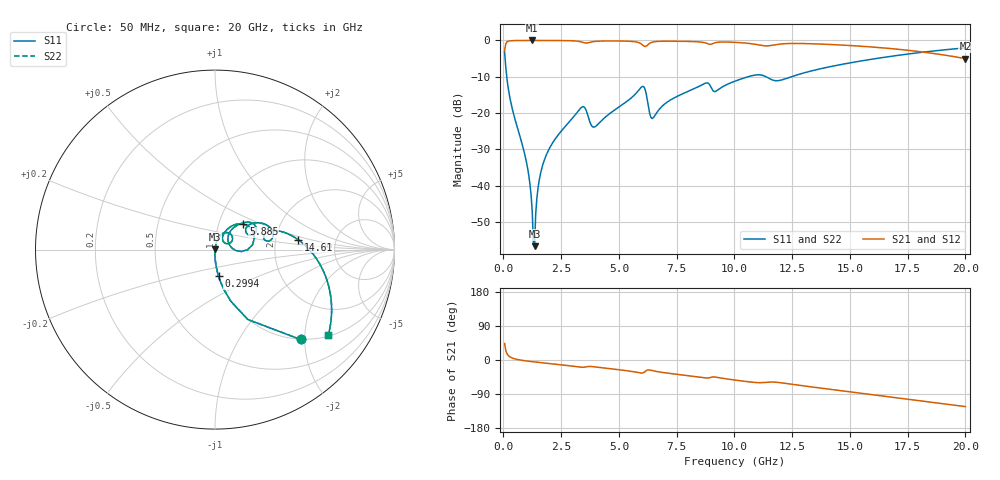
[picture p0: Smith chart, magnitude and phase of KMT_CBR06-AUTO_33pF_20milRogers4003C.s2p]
! Data measured by Modelithics Inc. support@modelithics.com 813-866-6335
! KEMET CBR06-AUTO 33pF, Pad Width= 0.851mm, Pad Length= 0.64mm, Pad Gap= 0.62mm, 20mil Rogers 4003C substrate Data, January 2022
# hz S ma R 50
! 2 Port Network Data from SP1.SP block
! freq  magS11  angS11  magS21  angS21  magS12  angS12  magS22  angS22
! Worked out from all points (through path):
!   401 points, 50 MHz to 20 GHz, reference 50 ohm
!   highest |S21| = -0.01 dB at 1.247 GHz (marker M1); lowest = -5.0 dB at 20 GHz (marker M2)
!   group delay of S21, straight-line fit = 17.1 ps
!   lowest |S11| = -56.6 dB at 1.347 GHz (marker M3), VSWR 1.00, Z = 50.1 + j0.129 ohm
!   |S11| at or under -10 dB: 143 MHz to 10.58 GHz (10.44 GHz wide, 195 % of centre); 11.37 GHz to 12.46 GHz (1.09 GHz wide, 9.15 % of centre)
!   |S22| runs from -56.6 to -2.1 dB; largest |S21 - S12| = 0
!   S11 on the Smith chart (normalised r, x): 50 MHz: 0.99, -1.91; 299.4 MHz: 0.99, -0.30; 5.885 GHz: 1.31, +0.39; 14.61 GHz: 2.68, +0.38; 20 GHz: 1.05, -2.63
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5e7  0.6914 -46.4  0.722 43.6  0.722 43.6  0.6914 -46.4
2.99375e8  0.1504 -82.4  0.9883 7.5  0.9883 7.5  0.1504 -82.4
9.97625e8  0.02103 -91.2  0.9992 -2.6  0.9992 -2.6  0.02103 -91.2
1.14725e9  0.01058 -90.7  0.9993 -3.7  0.9993 -3.7  0.01058 -90.7
1.247e9  0.004417 -86.9  0.9994 -4.4  0.9994 -4.4  0.004417 -86.9
1.34675e9  0.001479 60.4  0.9993 -5.1  0.9993 -5.1  0.001479 60.4
1.54625e9  0.01184 80.2  0.9992 -6.5  0.9992 -6.5  0.01184 80.2
1.8455e9  0.02612 79.7  0.9988 -8.4  0.9988 -8.4  0.02612 79.7
3.391625e9  0.1209 49.5  0.9497 -19.2  0.9497 -19.2  0.1209 49.5
3.94025e9  0.06443 44.0  0.968 -18.1  0.968 -18.1  0.06443 44.0
5.885375e9  0.2121 41.8  0.9257 -33.9  0.9257 -33.9  0.2121 41.8
6.084875e9  0.2291 16.5  0.8351 -32.7  0.8351 -32.7  0.2291 16.5
6.434e9  0.08433 23.0  0.9443 -27.8  0.9443 -27.8  0.08433 23.0
6.73325e9  0.1116 47.5  0.9722 -31.4  0.9722 -31.4  0.1116 47.5
8.678375e9  0.2528 36.0  0.9356 -46.7  0.9356 -46.7  0.2528 36.0
9.177125e9  0.199 30.6  0.9317 -45.1  0.9317 -45.1  0.199 30.6
1.0025e10  0.2754 32.9  0.9412 -53.0  0.9412 -53.0  0.2754 32.9
1.152125e10  0.298 9.1  0.8465 -58.3  0.8465 -58.3  0.298 9.1
1.336662e10  0.3833 15.2  0.8999 -71.3  0.8999 -71.3  0.3833 15.2
1.46135e10  0.4661 6.8  0.8652 -80.8  0.8652 -80.8  0.4661 6.8
1.670825e10  0.6001 -9.2  0.7762 -97.0  0.7762 -97.0  0.6001 -9.2
2e10  0.7897 -36.9  0.5613 -123.0  0.5613 -123.0  0.7897 -36.9
